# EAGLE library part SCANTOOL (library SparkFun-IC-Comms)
Multiprotocol OBD II to UART Interpreter, QFN Package This part, the STN1110, is a preprogrammed pic from ScanTool. Contact: vit@scantool.net Datasheet SparkFun Products SparkFun OBD-II UART (WIG-09555)
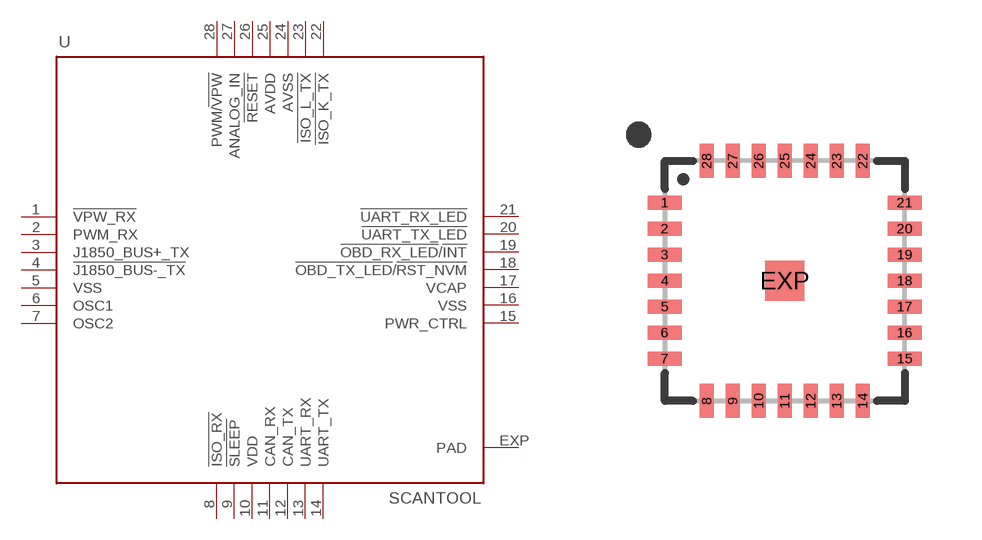
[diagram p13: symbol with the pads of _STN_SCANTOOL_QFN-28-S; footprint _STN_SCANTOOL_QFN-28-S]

Designator prefix U

## SCANTOOL (PROD_ID: IC-10017; VALUE: STN1110)  [_STN_SCANTOOL_QFN-28-S]
1  !VPW_RX  in
2  PWM_RX  in
3  J1850_BUS+_TX  out
4  !J1850_BUS-_TX  out
5  VSS  pwr
6  OSC1  in
7  OSC2  out
8  !ISO_RX  in
9  !SLEEP  in
10  VDD  pwr
11  CAN_RX  in
12  CAN_TX  out
13  UART_RX  in
14  UART_TX  out
15  PWR_CTRL  out
16  VSS  pwr
17  VCAP  pwr
18  !OBD_TX_LED!/!RST_NVM
19  !OBD_RX_LED!/!INT  out
20  !UART_TX_LED  out
21  !UART_RX_LED  out
22  !ISO_K_TX  out
23  !ISO_L_TX  out
24  AVSS  pwr
25  AVDD  pwr
26  !RESET  in
27  ANALOG_IN  in
28  PWM/!VPW  out
EXP  PAD  pas

## Footprint _STN_SCANTOOL_QFN-28-S (pad centres in mm)
Quad Flat No Leads Package Specifications: Pin count:28 Example device(s): SCANTOOL Change Log DateAuthorChange March 23, 2010joe@scantool.netAdded t-keepout layer. March 22,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
smd 0.85 x 0.35: 1 -3,1.95; 2 -3,1.3; 3 -3,0.65; 4 -3,0; 5 -3,-0.65; 6 -3,-1.3; 7 -3,-1.95; 15 3,-1.95; 16 3,-1.3; 17 3,-0.65; 18 3,0; 19 3,0.65; 20 3,1.3; 21 3,1.95
smd 0.35 x 0.85: 8 -1.95,-3; 9 -1.3,-3; 10 -0.65,-3; 11 0,-3; 12 0.65,-3; 13 1.3,-3; 14 1.95,-3; 22 1.95,3; 23 1.3,3; 24 0.65,3; 25 0,3; 26 -0.65,3; 27 -1.3,3; 28 -1.95,3
smd 1 x 1: EXP 0,0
